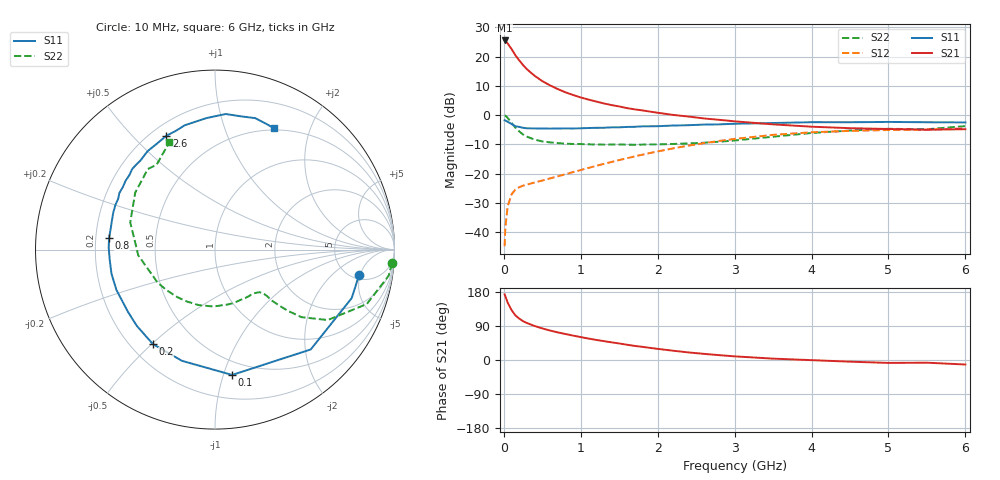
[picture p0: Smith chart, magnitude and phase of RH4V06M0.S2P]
! SIEMENS Small Signal Semiconductors
! BFR106
! Si NPN RF Bipolar Junction Transistor in SOT23
! VCE = 4 V  IC = 6 mA
! Common Emitter S-Parameters:  August  1996
# GHz  S  MA  R  50
!  f  S11  S21  S12  S22
! GHz  MAG  ANG  MAG  ANG  MAG  ANG  MAG  ANG
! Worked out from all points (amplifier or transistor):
!   36 points, 10 MHz to 6 GHz, reference 50 ohm
!   highest |S21| = 25.5 dB at 10 MHz (marker M1)
!   |S21| within 3 dB of that: start of sweep to 102 MHz
!   unconditionally stable (mu >= 1): 584.5 MHz to 2.03 GHz; 4.97 GHz to end of sweep
!   at 250 MHz: K = 0.56, MSG = 20.6 dB, |S12| = -24.1 dB
!   at 1.4 GHz: K = 1.12, MAG = 7.6 dB, |S12| = -16.0 dB
!   at 6 GHz: K = 1.02, MAG = -1.0 dB, |S12| = -4.5 dB
!   S11 on the Smith chart (normalised r, x): 10 MHz: 5.69, -4.80; 100 MHz: 0.39, -1.07; 200 MHz: 0.29, -0.50; 800 MHz: 0.26, +0.05; 2.6 GHz: 0.26, +0.63; 6 GHz: 0.48, +1.49
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0.01  0.815 -10.0  18.83 173.2  0.0058 86.2  0.9897 -4.4
0.02  0.8083 -19.5  18.48 168.0  0.0122 80.7  0.9781 -8.6
0.05  0.7707 -46.2  16.73 151.3  0.0277 67.3  0.8988 -19.7
0.1  0.7049 -82.2  13.46 131.8  0.0445 53.5  0.7407 -32.0
0.15  0.6465 -106.5  10.55 117.9  0.0536 45.5  0.6113 -38.0
0.2  0.6301 -123.3  8.614 109.3  0.0588 42.3  0.5281 -40.1
0.25  0.6084 -135.8  7.149 102.3  0.0625 40.6  0.4659 -41.2
0.3  0.5961 -144.5  6.08 97.6  0.0652 41.0  0.43 -41.8
0.4  0.5934 -157.7  4.697 89.8  0.0708 42.3  0.3823 -41.8
0.5  0.5922 -167.0  3.808 83.3  0.0767 45.2  0.3564 -42.4
0.6  0.5893 -174.7  3.224 77.8  0.0831 48.0  0.3424 -43.9
0.8  0.5941 173.8  2.457 68.6  0.0979 53.0  0.3256 -48.4
1.1  0.6027 160.3  1.843 56.6  0.1256 58.5  0.318 -57.8
1.3  0.6088 152.5  1.584 49.8  0.1474 60.5  0.3139 -65.0
1.6  0.6287 142.4  1.32 40.3  0.1838 61.6  0.3139 -77.5
2.2  0.6647 124.4  1.01 24.5  0.2708 57.9  0.3223 -106.5
2.6  0.6898 113.1  0.879 16.2  0.3323 52.4  0.338 -128.4
3.5  0.7341 93.8  0.696 3.6  0.4608 36.6  0.4285 -175.7
4.5  0.7564 78.9  0.599 -4.4  0.539 17.6  0.5461 144.5
5  0.766 73.0  0.58 -7.7  0.5572 9.6  0.5845 129.8
5.5  0.7562 67.5  0.564 -7.1  0.5664 5.6  0.5736 124.6
6  0.7516 64.0  0.575 -11.9  0.5945 -2.3  0.6499 113.0
